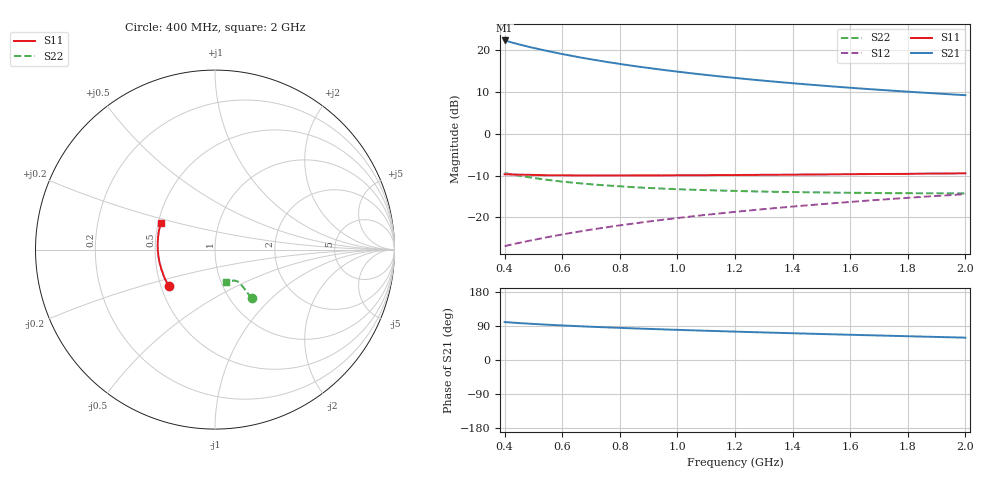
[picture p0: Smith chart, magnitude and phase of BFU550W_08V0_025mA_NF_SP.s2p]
! Filename:  P:\Prog\Test\Noise\ATS_data\Testdata_Net\06 Compressed Noise after Statistics\BFU550W_APM2013_11_D05_08p0V_025mA_NF_CM01_D.sf
! Date/Time: Tue 26/Mar/2013 16:25:25
! BFU550W_APM2013_11_D05_08p0V_1to35mA_NF_CM01_Bias8_R.sf
! Noise Parameter Data File
! BFU550W_APM2013_11_D05_08p0V_1to35mA_NF_CM01
! Date/time: Mon Mar 25 14:39:45 2013
! VAR V_out= 8.000000
! VAR I_out= 24.990000
! VAR V_in= 0.796000
! VAR I_in= 0.248850
! Device data file deembeded for feedlines and parallel
! Original file: \06 Compressed Noise after Statistics\BFU550W_APM2013_11_D05_08p0V_025mA_NF_CM01_R.sf
! Feed-files: PR019V01_070313_Feed1.s2p, PR019V01_070313_Feed2.s2p
! Parallel-file: PR019V01_070313_Par.s2p
# MHz S MA R 50
!  Freq-MHz  S11-mag  S11-arg  S21-mag  S21-arg  S12-mag  S12-arg  S22-mag  S22-arg
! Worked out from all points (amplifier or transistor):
!   37 points, 400 MHz to 2 GHz, reference 50 ohm
!   highest |S21| = 22.3 dB at 400 MHz (marker M1)
!   |S21| within 3 dB of that: start of sweep to 582.8 MHz
!   unconditionally stable (mu >= 1): 1.042 GHz to end of sweep
!   at 500 MHz: K = 0.91, MSG = 23.0 dB, |S12| = -25.4 dB
!   at 1.1 GHz: K = 1.00, MAG = 16.4 dB, |S12| = -19.4 dB
!   at 2 GHz: K = 1.00, MAG = 11.4 dB, |S12| = -14.5 dB
!   lowest NFmin = 1.06 dB at 440 MHz
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400  0.3271 -142.2  13.05 100.2  0.04518 67.5  0.3391 -52.8
420  0.326 -144.6  12.48 99.0  0.04688 67.8  0.3292 -53.0
440  0.3245 -146.6  11.96 98.0  0.04857 68.0  0.3195 -53.0
460  0.3236 -148.4  11.48 97.0  0.05028 68.3  0.311 -53.1
480  0.3226 -150.4  11.04 96.1  0.05197 68.6  0.3033 -53.2
500  0.3217 -152.3  10.63 95.2  0.05365 68.8  0.2959 -53.1
550  0.3185 -156.1  9.746 93.1  0.05802 69.3  0.2804 -53.1
600  0.3186 -159.7  8.982 91.2  0.06238 69.8  0.2672 -53.1
650  0.317 -162.8  8.327 89.4  0.06677 70.1  0.2573 -53.1
700  0.3172 -165.6  7.761 87.8  0.07123 70.3  0.2484 -53.3
750  0.3171 -168.2  7.27 86.3  0.07562 70.5  0.241 -53.4
800  0.3169 -170.8  6.836 84.8  0.0801 70.7  0.2351 -53.8
850  0.3176 -173.1  6.453 83.4  0.08451 70.7  0.2291 -53.8
950  0.3174 -177.0  5.804 80.8  0.09353 70.8  0.2206 -54.4
1050  0.3187 179.3  5.277 78.4  0.1026 70.7  0.2141 -55.4
1150  0.3207 175.8  4.839 76.0  0.1116 70.4  0.209 -56.4
1200  0.3206 174.4  4.651 74.9  0.1163 70.3  0.207 -57.1
1350  0.323 170.0  4.16 71.7  0.1299 69.7  0.2016 -58.9
1500  0.3255 165.8  3.768 68.6  0.1436 68.9  0.1987 -61.4
1650  0.3289 162.0  3.447 65.6  0.1573 68.0  0.1961 -63.8
1750  0.3307 159.8  3.267 63.7  0.1665 67.4  0.1944 -65.6
2000  0.3364 154.1  2.891 59.0  0.1893 65.7  0.1932 -70.9
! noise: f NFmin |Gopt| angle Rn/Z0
400  1.077  0.2997  -173.7  0.074
460  1.067  0.3085  -171.5  0.073
600  1.076  0.3113  -169.7  0.0755
800  1.143  0.3227  -165.5  0.0735
1000  1.15  0.3374  -161.4  0.0728
1200  1.201  0.3429  -157.6  0.077
1400  1.208  0.357  -153.3  0.0808
1600  1.234  0.3647  -151.5  0.0834
1800  1.267  0.3854  -146.8  0.088
2000  1.297  0.3878  -143.2  0.0956
